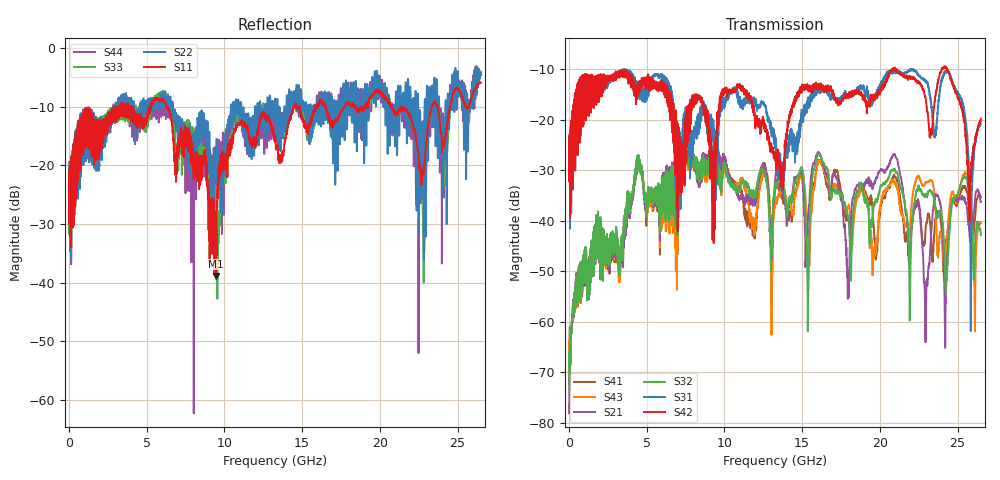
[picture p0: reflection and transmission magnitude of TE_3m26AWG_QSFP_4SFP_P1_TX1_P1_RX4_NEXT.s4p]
!Agilent Technologies,N5222A,MY51421691,A.10.00.00
!Agilent N5222A: A.10.00.00
!Date: Friday, January 30, 2015 12:34:46
!Correction: S11(Full 4 Port(1,2,3,4))
!S12(Full 4 Port(1,2,3,4))
!S13(Full 4 Port(1,2,3,4))
!S14(Full 4 Port(1,2,3,4))
!S21(Full 4 Port(1,2,3,4))
!S22(Full 4 Port(1,2,3,4))
!S23(Full 4 Port(1,2,3,4))
!S24(Full 4 Port(1,2,3,4))
!S31(Full 4 Port(1,2,3,4))
!S32(Full 4 Port(1,2,3,4))
!S33(Full 4 Port(1,2,3,4))
!S34(Full 4 Port(1,2,3,4))
!S41(Full 4 Port(1,2,3,4))
!S42(Full 4 Port(1,2,3,4))
!S43(Full 4 Port(1,2,3,4))
!S44(Full 4 Port(1,2,3,4))
!S4P File: Measurements: <S11,S12,S13,S14>,
!<S21,S22,S23,S24>,
!<S31,S32,S33,S34>,
!<S41,S42,S43,S44>:
# Hz S  dB  R 50.0
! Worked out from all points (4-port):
!   2650 points, 10 MHz to 26.5 GHz, reference 50 ohm
!   strongest paths, dB at 10 MHz, 6.63 GHz, 13.26 GHz, 19.88 GHz, 26.5 GHz:
!     S42: -25.0, -19.2, -26.9, -14.9, -19.8
!     S31: -24.8, -18.2, -24.4, -13.7, -20.8
!     S32: -67.0, -29.1, -33.3, -35.0, -42.8
!     S21: -78.1, -28.5, -31.9, -30.5, -36.2
!     S43: -63.7, -29.8, -36.1, -41.4, -40.4
!     S41: -64.4, -29.1, -34.0, -43.0, -35.3
!   lowest |S11| = -38.8 dB at 9.43 GHz (marker M1), VSWR 1.02, Z = 50.5 + j1.04 ohm
!   |S11| at or under -10 dB: start of sweep to 2.939 GHz; 6.342 GHz to 14.46 GHz (8.113 GHz wide, 78 % of centre); 21.35 GHz to 23.34 GHz (1.987 GHz wide, 8.89 % of centre)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
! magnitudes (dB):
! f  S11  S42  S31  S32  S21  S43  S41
! 10 MHz  -20.9  -25.0  -24.8  -67.0  -78.1  -63.7  -64.4
! 4.41 GHz  -11.6  -13.5  -13.5  -28.7  -28.6  -29.1  -29.1
! 9.43 GHz  -38.8  -24.4  -27.4  -29.4  -26.7  -29.6  -27.1
! 17.95 GHz  -9.2  -14.9  -15.0  -39.4  -50.8  -37.5  -39.6
! 20.96 GHz  -10.9  -9.8  -10.7  -29.7  -26.8  -32.5  -31.3
! 22.96 GHz  -16.7  -16.0  -12.3  -34.7  -56.9  -32.4  -41.0
! 26.5 GHz  -5.9  -19.8  -20.8  -42.8  -36.2  -40.4  -35.3
